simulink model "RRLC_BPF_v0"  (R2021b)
settings: Solver=VariableStepAuto  StartTime=0.0  StopTime=0.03  MaxStep=1e-4  RelTol=1e-3
libraries: fl_lib x8, nesl_utility x3

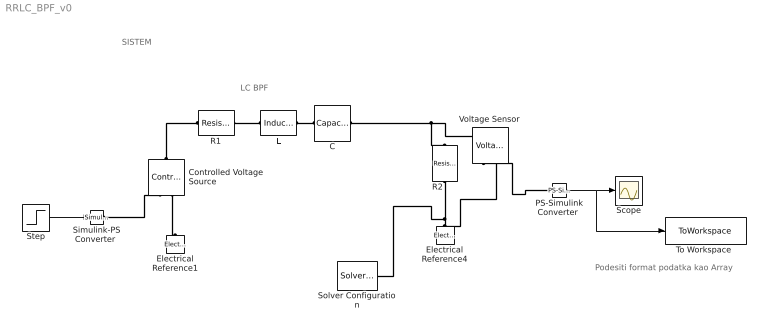
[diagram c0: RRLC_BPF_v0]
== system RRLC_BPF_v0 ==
  note: Podesiti format podatka kao Array
  note: SISTEM
  note: LC BPF
  C : fl_lib/Electrical/Electrical Elements/Capacitor  c=C_var F  r=1e-6 Ohm  g=0 1/Ohm  i_specify=off  i_priority=None  i=0 A  i_nominal_specify=off  i_nominal_unit=A  i_nominal_value=1  v_specify=off  v_priority=None  v=0 V  v_nominal_specify=off  v_nominal_unit=V  v_nominal_value=1  vc_specify=off  vc_priority=High  vc=0 V  vc_nominal_specify=off  vc_nominal_unit=V  vc_nominal_value=1
  "Controlled Voltage Source " : fl_lib/Electrical/Electrical Sources/Controlled Voltage Source
  Electrical Reference1 : fl_lib/Electrical/Electrical Elements/Electrical Reference
  Electrical Reference4 : fl_lib/Electrical/Electrical Elements/Electrical Reference
  L : fl_lib/Electrical/Electrical Elements/Inductor  l=1 H  r=0 Ohm  g=1e-9 1/Ohm  i_specify=off  i_priority=None  i=0 A  i_nominal_specify=off  i_nominal_unit=A  i_nominal_value=1  v_specify=off  v_priority=None  v=0 V  v_nominal_specify=off  v_nominal_unit=V  v_nominal_value=1  i_L_specify=off  i_L_priority=High  i_L=0 A  i_L_nominal_specify=off  i_L_nominal_unit=A  i_L_nominal_value=1
  "PS-Simulink Converter " : nesl_utility/PS-Simulink Converter  PhysicalDomain=network_engine_domain  SubClassName=ps_output  LeftPortType=input  RightPortType=output  PseudoPeriodic=off  Frequencies=[]  Unit=inherit  AffineConversion=off
  R1 : fl_lib/Electrical/Electrical Elements/Resistor  R=1 kOhm  i_specify=off  i_priority=None  i=0 A  i_nominal_specify=off  i_nominal_unit=A  i_nominal_value=1  v_specify=off  v_priority=None  v=0 V  v_nominal_specify=off  v_nominal_unit=V  v_nominal_value=1
  R2 : fl_lib/Electrical/Electrical Elements/Resistor  R=1 kOhm  i_specify=off  i_priority=None  i=0 A  i_nominal_specify=off  i_nominal_unit=A  i_nominal_value=1  v_specify=off  v_priority=None  v=0 V  v_nominal_specify=off  v_nominal_unit=V  v_nominal_value=1
  Scope : Scope
  "Simulink-PS Converter " : nesl_utility/Simulink-PS Converter  PhysicalDomain=network_engine_domain  SubClassName=ps_input  LeftPortType=input  RightPortType=output  PseudoPeriodic=off  Frequencies=[]  NoiseDistribution=none  NoiseParameters=[]  Unit=1  AffineConversion=off  FilteringAndDerivatives=provide  SimscapeFilterOrder=1  InputFilterTimeConstant=0.001  UdotUserProvided=0
  Solver Configuration : nesl_utility/Solver Configuration  PhysicalDomain=network_engine_domain  SubClassName=solver  LeftPortType=input  RightPortType=generic  Tones=[]  Harmonics=[]  SimulateNoise=off  Profile=off  UseLocalSampling=off  EnableSwitchedLinearOptims=on  FrequencyDomain=off  UseCCode=off  RelTol=0.001  AbsTol=1e-06  MinStep=1e-09  ToWorkspace=off  RevertToSquareIcSolve=off  NumHomotopyIterations=100  PhasorMode=off  PhasorModeNumHarmonics=1  DoDC=off  ResidualTolerance=1e-09  UseLocalSolver=off  LocalSolverChoice=NE_BACKWARD_EULER_ADVANCER  LocalSolverSampleTime=0.001  DoFixedCost=off  MaxNonlinIter=3  MaxModeIter=2  ComputeImpulses=off  ImpulseIterations=2  LinearAlgebra=auto  EquationFormulation=NE_TIME_EF  DelaysMemoryBudget=1024  AutomaticFiltering=on  FilteringTimeConstant=0.001  PartitionStorageMethod=AS_NEEDED  PartitionMemoryBudget=1024  PartitionMethod=ROBUST
  Step : Step  Before=0.01  SampleTime=0
  "To Workspace " : ToWorkspace  VariableName=vR2  SampleTime=-1
  Voltage Sensor : fl_lib/Electrical/Electrical Sensors/Voltage Sensor
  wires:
  "PS-Simulink Converter "/1 -> "To Workspace "/1, Scope/1
  Step/1 -> "Simulink-PS Converter "/1
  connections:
  L/RConn1 -- C/LConn1
  C/RConn1 -- R2/LConn1 -- Voltage Sensor/LConn1
  R1/RConn1 -- L/LConn1
  Electrical Reference4/LConn1 -- Voltage Sensor/RConn2 -- Solver Configuration/RConn1 -- R2/RConn1
  "PS-Simulink Converter "/LConn1 -- Voltage Sensor/RConn1
  "Simulink-PS Converter "/RConn1 -- "Controlled Voltage Source "/RConn1
  "Controlled Voltage Source "/LConn1 -- R1/LConn1
  "Controlled Voltage Source "/RConn2 -- Electrical Reference1/LConn1
